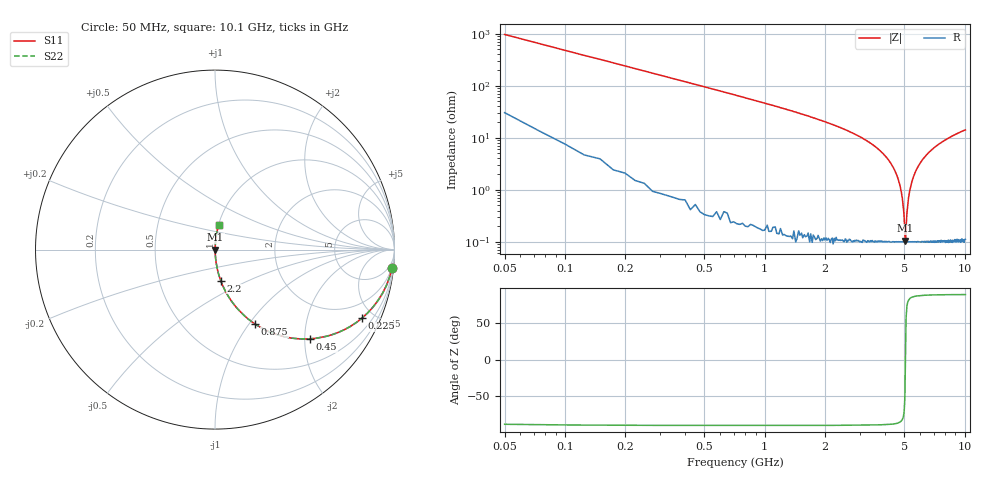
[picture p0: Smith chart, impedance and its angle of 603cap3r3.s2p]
! AVX Thin Film Operation		Date: November 2004
! Description: Accu-P® Series, Thin Film, SMD, RF Capacitor
! Part Number: 06035J3R3ABT
! 50 MHz  -  10.05 GHz
! Serial Measurements
# hz S db R 50
!	S11		S21		S12		S22
!	dB	Phase	dB	Phase	dB	Phase	dB	Phase
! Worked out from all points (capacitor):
!   400 points, 50 MHz to 10.1 GHz, reference 50 ohm
!   read as one part in series: C = 3.3 pF near 100 MHz
!   lowest |Z| = 105 mohm at 5.05 GHz (marker M1)
!   series resonance near 5.06 GHz, so ESL is about 300 pH
!   S11 on the Smith chart (normalised r, x): 50 MHz: 2, -19; 225 MHz: 1.03, -4.27; 450 MHz: 1.01, -2.13; 875 MHz: 1.00, -1.07; 2.2 GHz: 1.00, -0.36; 10.1 GHz: 1.00, +0.28
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5e7  -0.08 -5.9  -19.80 82.3  -19.80 82.3  -0.08 -5.9
1.25e8  -0.31 -14.5  -12.00 74.8  -12.00 74.8  -0.31 -14.5
2.25e8  -0.88 -25.0  -7.49 64.6  -7.49 64.6  -0.88 -25.0
4.5e8  -2.77 -43.1  -3.30 46.6  -3.30 46.6  -2.77 -43.1
8.75e8  -6.54 -61.7  -1.11 28.1  -1.11 28.1  -6.54 -61.7
1.73e9  -12.40 -75.9  -0.27 13.9  -0.27 13.9  -12.40 -75.9
2.2e9  -15.10 -79.6  -0.14 10.1  -0.14 10.1  -15.10 -79.6
3.4e9  -22.20 -84.8  -0.04 4.4  -0.04 4.4  -22.20 -84.8
4.28e9  -29.80 -86.4  -0.01 1.8  -0.01 1.8  -29.80 -86.4
4.68e9  -36.40 -85.3  -0.01 0.9  -0.01 0.9  -36.40 -85.3
4.93e9  -45.70 -78.6  -0.01 0.3  -0.01 0.3  -45.70 -78.6
4.98e9  -49.60 -72.3  -0.01 0.2  -0.01 0.2  -49.60 -72.3
5.05e9  -59.60 -17.3  -0.01 0.0  -0.01 0.0  -59.60 -17.3
5.08e9  -58.60 32.2  -0.01 -0.0  -0.01 -0.0  -58.60 32.2
5.1e9  -54.60 57.4  -0.01 -0.1  -0.01 -0.1  -54.60 57.4
5.15e9  -49.00 73.5  -0.01 -0.2  -0.01 -0.2  -49.00 73.5
5.2e9  -45.40 79.0  -0.01 -0.3  -0.01 -0.3  -45.40 79.0
5.45e9  -36.90 85.2  -0.01 -0.8  -0.01 -0.8  -36.90 85.2
5.9e9  -30.60 86.4  -0.01 -1.7  -0.01 -1.7  -30.60 86.4
6.75e9  -25.10 85.8  -0.02 -3.2  -0.02 -3.2  -25.10 85.8
8.43e9  -19.90 83.6  -0.05 -5.8  -0.05 -5.8  -19.90 83.6
1.01e10  -17.10 81.5  -0.10 -8.0  -0.10 -8.0  -17.10 81.5
